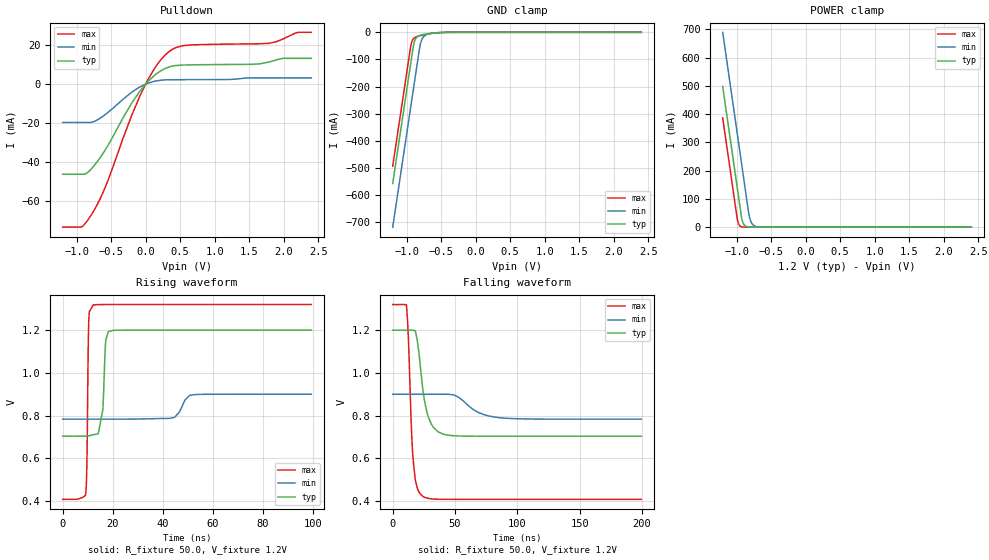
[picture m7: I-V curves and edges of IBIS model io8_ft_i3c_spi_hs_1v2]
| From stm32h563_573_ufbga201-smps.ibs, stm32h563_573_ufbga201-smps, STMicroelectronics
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[Model]   io8_ft_i3c_spi_hs_1v2
Model_type I/O_open_drain
Polarity   Non-Inverting
Enable   Active-Low
| CAP_THRESHOLD on pad IOFT is "UDTCAPC" :
| Rising=20.0% of vddiom   Falling=80.0% of vddiom
| C_comp min and max val. don't necessarily correlate with the min and max pvt
| but are the smallest and greatest pad capacitance found.
| var   typ   min   max
C_comp   3.41735pF  3.39635pF  3.42855pF
|C_comp_pulldown   3.41735pF  3.39635pF  3.42855pF
Vinl = 450.0mV
Vinh = 660.0mV
Vmeas = 600.0mV   | Reference voltage for timing measurements
Cref  = 50.0pF   | Timing specification test load capacitance value
Rref  = 1.0MOhm   | Timing specification test load resistance value
Vref  = 660.0mV   | Timing specification test load voltage
[Model Spec]
| TIME_THRESHOLD on pin ZII2CV11 is "CMOS" :
| Rising=40.0% of vdd   Falling=60.0% of vdd
Vinl 447.80000mV 344.80000mV 489.80000mV
Vinh 733.20000mV 535.20000mV 813.20000mV
| variable   typ   min   max
[Temperature Range] 25.0 125.0 -40.0
| variable   typ   min   max
[Voltage Range] 1.2V 900.0mV 1.32V
| variable   typ   min   max
[POWER Clamp Reference] 1.2V 900.0mV 1.32V
| variable   typ   min   max
[GND Clamp Reference] 0V 0V 0V
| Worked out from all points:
|   slope of the pulldown table from 0 to 0.18 V, typ, clamps not added: 30.6 ohm
|   GND clamp passes 1 mA (typ) near -0.52 V on its own axis
|   POWER clamp passes 1 mA (typ) near -0.84 V on its own axis
|   rising waveform, R_fixture 50.0, V_fixture 1.2V: 20-80 % time 1.29ns typ, 3.34ns min, 533ps max; typ from 0.704 V to 1.2 V
|   falling waveform, R_fixture 50.0, V_fixture 1.2V: 20-80 % time 7.21ns typ, 17.2ns min, 3.72ns max; typ from 1.2 V to 0.704 V
[POWER Clamp]
-1.2V     497.8mA    689.2mA    386.5mA
-990mV    140.8mA    332.2mA    29.53mA
-980mV    123.8mA    315.2mA    17.95mA
-960mV    89.81mA    281.2mA    6.634mA
-930mV    38.81mA    230.2mA    1.49mA
-900mV    12.07mA    179.2mA    334.8uA
-870mV    3.756mA    128.2mA    75.22uA
-820mV    536.4uA    44.98mA    6.246uA
-790mV    166.9uA    18.76mA    1.403uA
-750mV    35.18uA    5.846mA    191.8nA
-590mV    70.09nA    55uA       165.5pA
2.4V      0A         0A         0A
[GND Clamp]
-1.2V     -558.2mA   -719mA     -494.1mA
-940mV    -116.2mA   -277mA     -52.06mA
-930mV    -99.19mA   -260mA     -39.94mA
-900mV    -49.1mA    -209mA     -23.76mA
-880mV    -30.14mA   -175mA     -19.6mA
-850mV    -17.82mA   -124mA     -16.09mA
-810mV    -11.73mA   -56.78mA   -12.91mA
-780mV    -9.444mA   -28.21mA   -10.92mA
-740mV    -7.291mA   -13.16mA   -8.574mA
-640mV    -3.573mA   -4.171mA   -3.954mA
-380mV    -61.75uA   -230.3uA   -20.32uA
2.4V      3.863nA    718.4nA    150.6pA
| variable   typ   min   max
[Pullup Reference] 1.2V 900.0mV 1.32V
| variable   typ   min   max
[Pulldown Reference] 0V 0V 0V
[Pulldown]
-1.2V     -46.17mA   -19.62mA   -73.27mA
-930mV    -46.17mA   -19.62mA   -73.18mA
-770mV    -42.8mA    -19.41mA   -66.04mA
-570mV    -32.88mA   -15.18mA   -51.58mA
-200mV    -9.658mA   -4.084mA   -15.89mA
-80mV     -3.488mA   -1.363mA   -5.887mA
120mV     4.232mA    1.387mA    7.501mA
340mV     8.782mA    2.251mA    16.66mA
540mV     9.805mA    2.305mA    19.74mA
1.79V     11.33mA    3.206mA    20.93mA
2.2V      13.23mA    3.206mA    26.48mA
2.4V      13.23mA    3.206mA    26.56mA
[Ramp]
dV/dt_r 297.79741mV/1.02425ns 69.90249mV/3.04456ns 547.13371mV/531.64653ps
dV/dt_f 297.80516mV/7.12458ns 69.9221mV/16.94277ns 547.13942mV/3.65468ns
R_load = 50.0
| Removed startup time: 0s 0s 0s  .
| Removed end time: 99.4ns.
[Rising Waveform]
R_fixture   = 50.0
V_fixture   = 1.2V
V_fixture_min = 900.0mV
V_fixture_max = 1.32V
0s        703.7mV    783.5mV    408.1mV
9.15ns    704mV      783.5mV    429.9mV
9.65ns    704.3mV    783.5mV    563.8mV
10.2ns    705mV      783.5mV    1.119V
10.45ns   705.4mV    783.5mV    1.251V
12.2ns    710.2mV    783.5mV    1.318V
16.05ns   826.7mV    783.5mV    1.32V
17.15ns   1.142V     783.5mV    1.32V
18.25ns   1.193V     783.5mV    1.32V
99.4ns    1.2V       900mV      1.32V
| Removed startup time: 0s 0s 0s  .
| Removed end time: 199.4ns.
[Falling Waveform]
R_fixture   = 50.0
V_fixture   = 1.2V
V_fixture_min = 900.0mV
V_fixture_max = 1.32V
0s        1.2V       900mV      1.32V
11ns      1.2V       900mV      1.318V
12.4ns    1.2V       900mV      1.186V
16.25ns   1.2V       900mV      601.8mV
19.85ns   1.146V     900mV      458.8mV
23.95ns   933.2mV    900mV      423mV
31.15ns   758.1mV    900.1mV    410.2mV
40.7ns    713mV      900mV      408.3mV
82.3ns    703.7mV    792.8mV    408.1mV
199.4ns   703.7mV    783.5mV    408.1mV
